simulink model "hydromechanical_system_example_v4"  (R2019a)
settings: Solver=VariableStepAuto  StartTime=0.0  StopTime=30  RelTol=1e-3
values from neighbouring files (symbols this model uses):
  A_B = 5*10^-4    (= 0.0005)    [codehydromechanical_system_example_v4.m]
  B = 1000    [codehydromechanical_system_example_v4.m]
  M = 100    [codehydromechanical_system_example_v4.m]
  R1 = 7*10^-6    (= 7e-06)    [codehydromechanical_system_example_v4.m]
  Vi = 0.001    [codehydromechanical_system_example_v4.m]

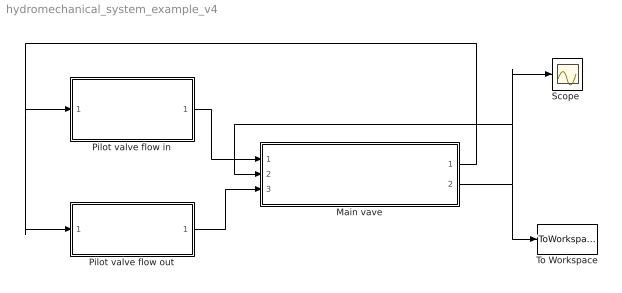
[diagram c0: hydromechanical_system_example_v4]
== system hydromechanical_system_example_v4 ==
  Main vave : Subsystem
  Pilot valve flow in : Subsystem
  Pilot valve flow out : Subsystem
  "Scope " : Scope
  To Workspace : ToWorkspace  VariableName=x_sim  SaveFormat=Timeseries  SampleTime=0.015
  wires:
  Main vave/1(Pc) -> Pilot valve flow out/1(Pc), Pilot valve flow in/1(Pc)
  Main vave/2(x) -> To Workspace/1, "Scope "/1, Main vave/2("x ")
  Pilot valve flow in/1(Qin) -> Main vave/1(Q_in)
  Pilot valve flow out/1(Qout) -> Main vave/3(Q_out)

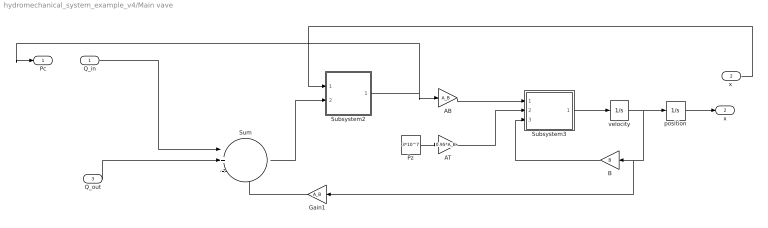
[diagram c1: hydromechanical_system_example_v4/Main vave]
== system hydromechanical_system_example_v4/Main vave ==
  Q_in : Inport
  "x " : Inport  Port=2
  Q_out : Inport  Port=3
  AB : Gain  Gain=A_B
  AT : Gain  Gain=0.95*A_B
  B : Gain  Gain=B
  Gain1 : Gain  Gain=A_B
  Pz : Constant  Value=3*10^7
  Subsystem2 : Subsystem
  Subsystem3 : Subsystem
  Sum : Sum  Inputs=|+--
  position : Integrator
  velocity : Integrator
  Pc : Outport
  x : Outport  Port=2
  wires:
  velocity/1 -> Gain1/1, B/1, position/1
  AT/1 -> Subsystem3/2(AT*Pc)
  Subsystem2/1(Pc) -> Pc/1, AB/1
  AB/1 -> Subsystem3/1(AB*Pc)
  Subsystem3/1("\\ddot{x} ") -> velocity/1
  B/1 -> Subsystem3/3("B\\dot{x}")
  Pz/1 -> AT/1
  Sum/1 -> Subsystem2/2(Q_total)
  Gain1/1 -> Sum/3
  Q_out/1 -> Sum/2
  position/1 -> x/1
  Q_in/1 -> Sum/1
  "x "/1 -> Subsystem2/1(AB*x)

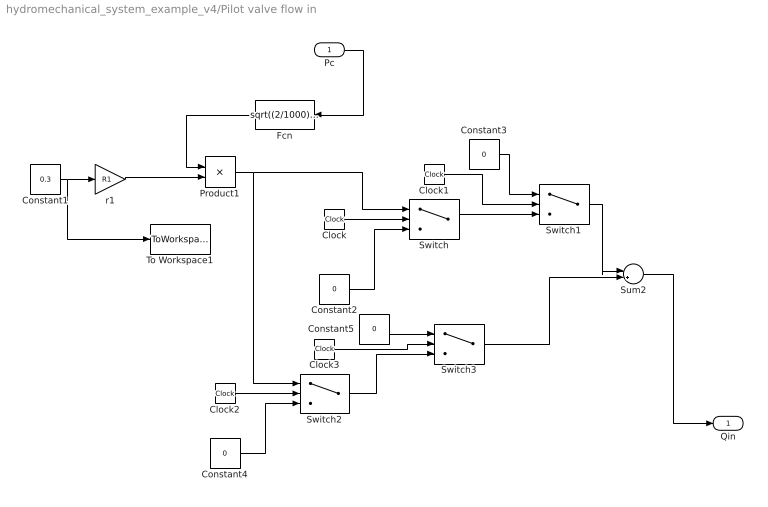
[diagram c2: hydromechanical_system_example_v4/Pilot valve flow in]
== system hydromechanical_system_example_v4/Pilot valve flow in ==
  Pc : Inport
  Clock{,1..3} (4 alike) : Clock
  Constant1 : Constant  Value=0.3
  Constant{2..5} (4 alike) : Constant  Value=0
  Fcn : Fcn  Expr=sqrt((2/1000)*(3*10^7-u))
  Product1 : Product
  Sum2 : Sum  Inputs=|++
  Switch : Switch  Criteria=u2 > Threshold  Threshold=2
  Switch1 : Switch  Criteria=u2 > Threshold  Threshold=4
  Switch2 : Switch  Criteria=u2 > Threshold  Threshold=15
  Switch3 : Switch  Criteria=u2 > Threshold  Threshold=18
  To Workspace1 : ToWorkspace  VariableName=v1_sim  SaveFormat=Timeseries  SampleTime=0.015
  r1 : Gain  Gain=R1
  Qin : Outport
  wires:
  Constant5/1 -> Switch3/1
  Fcn/1 -> Product1/1
  Constant1/1 -> To Workspace1/1, r1/1
  Product1/1 -> Switch2/1, Switch/1
  Clock2/1 -> Switch2/2
  Constant3/1 -> Switch1/1
  Switch3/1 -> Sum2/2
  Clock/1 -> Switch/2
  Constant2/1 -> Switch/3
  Switch1/1 -> Sum2/1
  Clock3/1 -> Switch3/2
  Clock1/1 -> Switch1/2
  Switch/1 -> Switch1/3
  Constant4/1 -> Switch2/3
  Switch2/1 -> Switch3/3
  r1/1 -> Product1/2
  Sum2/1 -> Qin/1
  Pc/1 -> Fcn/1

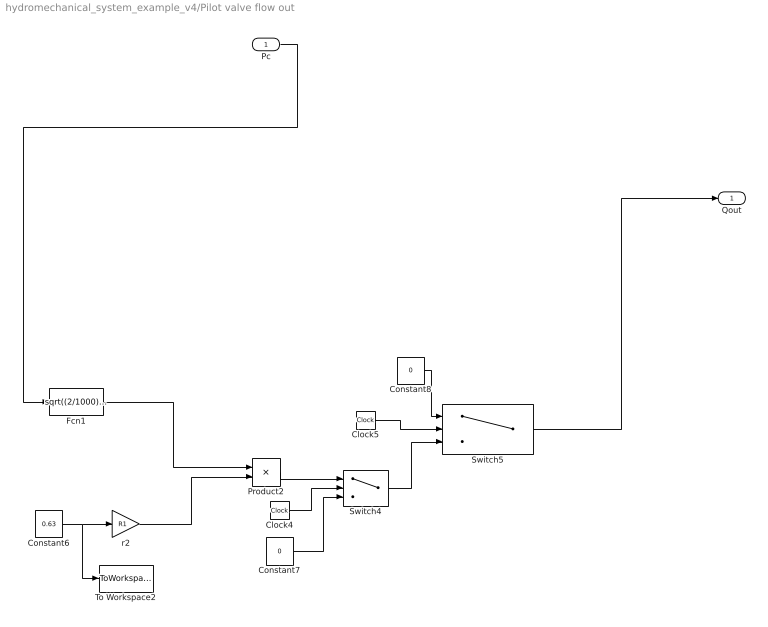
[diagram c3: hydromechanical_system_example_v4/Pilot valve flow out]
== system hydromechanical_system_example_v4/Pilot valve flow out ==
  Pc : Inport
  Clock4 : Clock
  Clock5 : Clock
  Constant6 : Constant  Value=0.63
  Constant7 : Constant  Value=0
  Constant8 : Constant  Value=0
  Fcn1 : Fcn  Expr=sqrt((2/1000)*u)
  Product2 : Product
  Switch4 : Switch  Criteria=u2 > Threshold  Threshold=23
  Switch5 : Switch  Criteria=u2 > Threshold  Threshold=23.51
  To Workspace2 : ToWorkspace  VariableName=v2_sim  SaveFormat=Timeseries  SampleTime=0.015
  r2 : Gain  Gain=R1
  Qout : Outport
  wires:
  Product2/1 -> Switch4/1
  Clock4/1 -> Switch4/2
  r2/1 -> Product2/2
  Constant8/1 -> Switch5/1
  Switch4/1 -> Switch5/3
  Constant7/1 -> Switch4/3
  Constant6/1 -> To Workspace2/1, r2/1
  Clock5/1 -> Switch5/2
  Fcn1/1 -> Product2/1
  Pc/1 -> Fcn1/1
  Switch5/1 -> Qout/1

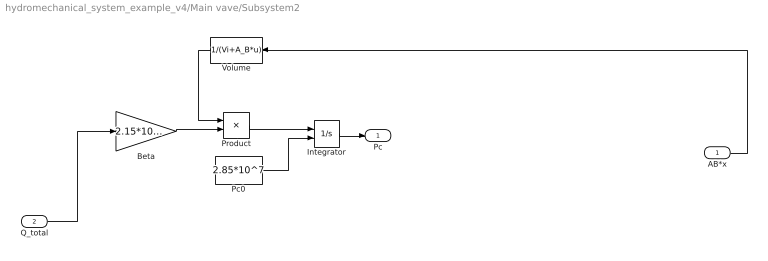
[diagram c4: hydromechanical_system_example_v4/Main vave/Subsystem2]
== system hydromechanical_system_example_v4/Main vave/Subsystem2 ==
  AB*x : Inport
  Q_total : Inport  Port=2
  Beta : Gain  Gain=2.15*10^9
  Integrator : Integrator  InitialConditionSource=external
  Pc0 : Constant  Value=2.85*10^7
  Product : Product
  Volume : Fcn  Expr=1/(Vi+A_B*u)
  Pc : Outport
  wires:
  Integrator/1 -> Pc/1
  Product/1 -> Integrator/1
  Volume/1 -> Product/1
  Pc0/1 -> Integrator/2
  Beta/1 -> Product/2
  Q_total/1 -> Beta/1
  AB*x/1 -> Volume/1

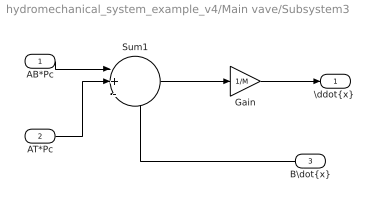
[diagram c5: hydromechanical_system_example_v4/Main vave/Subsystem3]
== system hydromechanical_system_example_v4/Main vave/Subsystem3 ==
  AB*Pc : Inport
  AT*Pc : Inport  Port=2
  "B\\dot{x}" : Inport  Port=3
  Gain : Gain  Gain=1/M
  Sum1 : Sum  Inputs=|+--
  "\\ddot{x} " : Outport
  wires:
  Gain/1 -> "\\ddot{x} "/1
  Sum1/1 -> Gain/1
  "B\\dot{x}"/1 -> Sum1/3
  AT*Pc/1 -> Sum1/2
  AB*Pc/1 -> Sum1/1
